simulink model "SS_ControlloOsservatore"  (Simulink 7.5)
settings: Solver=FixedStepDiscrete  StartTime=0.0  StopTime=10.0  FixedStep=Ts  RelTol=1e-3
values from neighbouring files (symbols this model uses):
  As1 = 1    [TSC160720ProvaMatlab.m]
  As2 = 2    [TSC160720ProvaMatlab.m]
  Kff = -inv(Cz*inv(Az-Bz*K-eye(n))*Bz)    [TSC160720ProvaMatlab.m]
  L = -acker(Az',Cz',[0 0 0])'    [TSC160720ProvaMatlab.m]
  ts1 = 0    [TSC160720ProvaMatlab.m]
  ts2 = 5    [TSC160720ProvaMatlab.m]
  X0 = [0, 0, 0]'    [TSC160720ProvaMatlab.m]
undefined symbols (not defined in the file or in its folder): Az, Bz, Cz, K
libraries: simulink x2

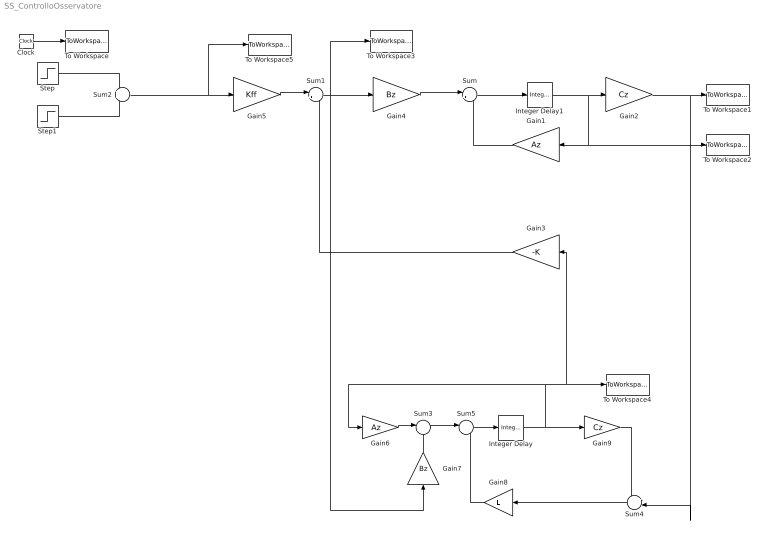
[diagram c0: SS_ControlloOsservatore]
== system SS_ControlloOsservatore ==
  Clock : Clock
  Gain1 : Gain  Gain=Az  Multiplication=Matrix(K*u)
  Gain2 : Gain  Gain=Cz  Multiplication=Matrix(K*u)
  Gain3 : Gain  Gain=-K  Multiplication=Matrix(K*u)
  Gain4 : Gain  Gain=Bz  Multiplication=Matrix(K*u)
  Gain5 : Gain  Gain=Kff  Multiplication=Matrix(K*u)
  Gain6 : Gain  Gain=Az  Multiplication=Matrix(K*u)
  Gain7 : Gain  Gain=Bz  Multiplication=Matrix(K*u)
  Gain8 : Gain  Gain=L  Multiplication=Matrix(K*u)
  Gain9 : Gain  Gain=Cz  Multiplication=Matrix(K*u)
  Integer Delay : simulink/Discrete/Integer Delay  vinit=[0 0 0]'  samptime=Ts  NumDelays=1
  Integer Delay1 : simulink/Discrete/Integer Delay  vinit=X0  samptime=Ts  NumDelays=1
  Step : Step  Time=ts1  After=As1  SampleTime=0
  Step1 : Step  Time=ts2  After=As2  SampleTime=0
  Sum{,1,3,5} (4 alike) : Sum  Inputs=|++
  Sum2 : Sum
  Sum4 : Sum  Inputs=+-
  To Workspace : ToWorkspace  VariableName=time  SampleTime=-1  SaveFormat=Array
  To Workspace1 : ToWorkspace  VariableName=y  SampleTime=-1  SaveFormat=Array
  To Workspace2 : ToWorkspace  VariableName=X  SampleTime=-1  SaveFormat=Array
  To Workspace3 : ToWorkspace  VariableName=u  SampleTime=-1  SaveFormat=Array
  To Workspace4 : ToWorkspace  VariableName=Xs  SampleTime=-1  SaveFormat=Array
  To Workspace5 : ToWorkspace  VariableName=yref  SampleTime=-1  SaveFormat=Array
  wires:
  Gain1/1 -> Sum/2
  Sum/1 -> Integer Delay1/1
  Integer Delay1/1 -> Gain2/1, Gain1/1, To Workspace2/1
  Gain4/1 -> Sum/1
  Clock/1 -> To Workspace/1
  Gain6/1 -> Sum3/1
  Integer Delay/1 -> Gain9/1, Gain6/1, Gain3/1, To Workspace4/1
  Gain7/1 -> Sum3/2
  Sum4/1 -> Gain8/1
  Gain9/1 -> Sum4/1
  Gain8/1 -> Sum5/2
  Sum3/1 -> Sum5/1
  Sum5/1 -> Integer Delay/1
  Gain5/1 -> Sum1/1
  Sum1/1 -> Gain4/1, To Workspace3/1, Gain7/1
  Gain3/1 -> Sum1/2
  Step/1 -> Sum2/1
  Step1/1 -> Sum2/2
  Sum2/1 -> To Workspace5/1, Gain5/1
  Gain2/1 -> Sum4/2, To Workspace1/1
